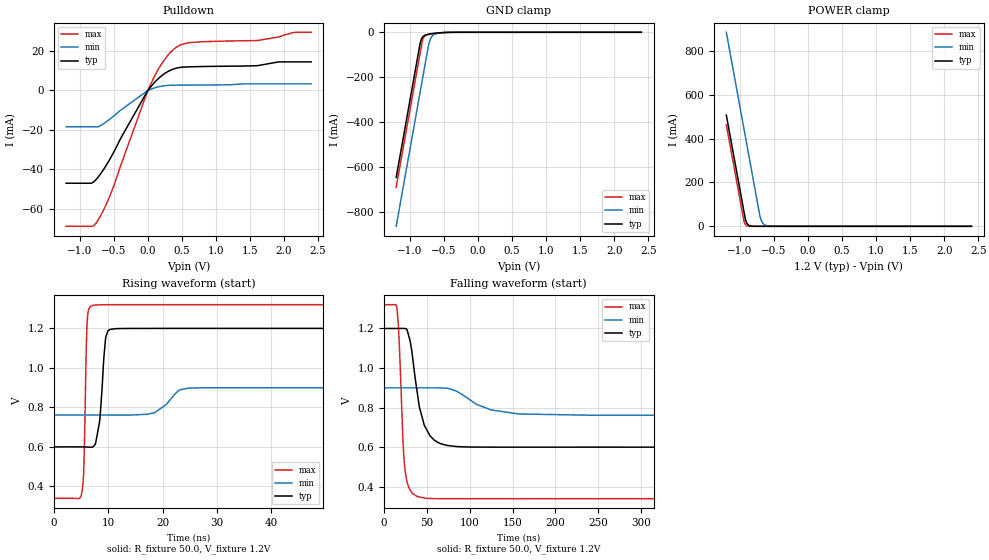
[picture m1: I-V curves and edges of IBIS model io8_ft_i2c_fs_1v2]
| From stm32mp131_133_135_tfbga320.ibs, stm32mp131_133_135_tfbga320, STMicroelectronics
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|   io8_ft_i2c_fs_1v2
[Model]   io8_ft_i2c_fs_1v2
Model_type I/O_open_drain
Polarity   Non-Inverting
Enable   Active-Low
| CAP_THRESHOLD on pad IOFT is "UDTCAPC" :
| Rising=20.0% of vddiom   Falling=80.0% of vddiom
| C_comp min and max val. don't necessarily correlate with the min and max pvt
| but are the smallest and greatest pad capacitance found.
| var   typ   min   max
C_comp   1.36950pF  1.28335pF  1.45130pF
Vinl = 360.0mV
Vinh = 840.0mV
Vmeas = 600.0mV   | Reference voltage for timing measurements
Cref  = 100.0nF   | Timing specification test load capacitance value
Rref  = 1.0kOhm   | Timing specification test load resistance value
Vref  = 600.1mV   | Timing specification test load voltage
[Model Spec]
| TIME_THRESHOLD on pin ZIV11 is "CMOS" :
| Rising=40.0% of vdd   Falling=60.0% of vdd
Vinl 465.80000mV 358.80000mV 518.80000mV
Vinh 741.20000mV 543.20000mV 820.20000mV
| variable   typ   min   max
[Temperature Range] 25.0 140.0 -40.0
| variable   typ   min   max
[Voltage Range] 1.2V 900.0mV 1.32V
| variable   typ   min   max
[POWER Clamp Reference] 1.2V 900.0mV 1.32V
| variable   typ   min   max
[GND Clamp Reference] 0V 0V 0V
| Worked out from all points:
|   slope of the pulldown table from 0 to 0.18 V, typ, clamps not added: 26.5 ohm
|   GND clamp passes 1 mA (typ) near -0.49 V on its own axis
|   POWER clamp passes 1 mA (typ) near -0.83 V on its own axis
|   rising waveform, R_fixture 50.0, V_fixture 1.2V: 20-80 % time 927ps typ, 3.09ns min, 434ps max; typ from 0.6 V to 1.2 V
|   falling waveform, R_fixture 50.0, V_fixture 1.2V: 20-80 % time 13.8ns typ, 35.7ns min, 5.62ns max; typ from 1.2 V to 0.6 V
[POWER Clamp]
-1.2V     507mA      884.8mA    462.5mA
-950mV    82mA       459.8mA    37.51mA
-930mV    48mA       425.8mA    13.86mA
-910mV    22.04mA    391.8mA    5.123mA
-890mV    10.12mA    357.8mA    1.893mA
-870mV    4.646mA    323.8mA    699.7uA
-710mV    9.171uA    51.95mA    243.5nA
-680mV    2.852uA    22.37mA    54.74nA
-650mV    886.6nA    9.63mA     12.33nA
-600mV    125.8nA    2.365mA    1.054nA
-490mV    1.049nA    108uA      41.48pA
2.4V      0A         0A         0A
[GND Clamp]
-1.2V     -646.3mA   -864.2mA   -690.1mA
-850mV    -51.35mA   -269.2mA   -95.05mA
-840mV    -39.26mA   -252.2mA   -78.05mA
-820mV    -24.85mA   -218.2mA   -44.05mA
-800mV    -17.5mA    -184.2mA   -25.22mA
-770mV    -12.13mA   -133.2mA   -15.02mA
-720mV    -8.143mA   -50.86mA   -9.665mA
-690mV    -6.656mA   -25.2mA    -7.855mA
-660mV    -5.424mA   -13.63mA   -6.324mA
-570mV    -2.602mA   -3.787mA   -2.765mA
-350mV    -41.28uA   -263.5uA   -8.566uA
2.4V      4.788nA    1.261uA    272.6pA
| variable   typ   min   max
[Pullup Reference] 1.2V 900.0mV 1.32V
| variable   typ   min   max
[Pulldown Reference] 0V 0V 0V
[Pulldown]
-1.2V     -47.11mA   -18.46mA   -68.98mA
-810mV    -46.78mA   -18.46mA   -68.93mA
-730mV    -44.02mA   -18.46mA   -65.79mA
-630mV    -39.07mA   -16.4mA    -59.3mA
-530mV    -33.22mA   -13.8mA    -51.19mA
0V        0A         0A         1fA
200mV     7.375mA    2.155mA    13.36mA
390mV     11.04mA    2.691mA    21.16mA
600mV     11.99mA    2.746mA    24.23mA
1.61V     12.59mA    3.342mA    25.35mA
2.15V     14.51mA    3.342mA    29.49mA
2.4V      14.51mA    3.342mA    29.54mA
[Ramp]
dV/dt_r 359.77616mV/926.94531ps 83.02607mV/3.08575ns 587.93904mV/432.99808ps
dV/dt_f 359.70168mV/13.79478ns 83.0117mV/35.69932ns 587.93923mV/5.62319ns
R_load = 50.0
| Removed startup time: 0s 0s 0s  .
| Removed end time: 2.1994us.
[Rising Waveform]
R_fixture   = 50.0
V_fixture   = 1.2V
V_fixture_min = 900.0mV
V_fixture_max = 1.32V
0s        600.4mV    761.6mV    340.1mV
5.1ns     600.3mV    761.6mV    362.6mV
5.5ns     600.2mV    761.6mV    474.1mV
6.2ns     599.2mV    761.6mV    1.261V
7.7ns     620.6mV    761.6mV    1.318V
8.8ns     866.8mV    761.6mV    1.319V
9.9ns     1.184V     761.5mV    1.32V
14.2ns    1.2V       761.5mV    1.32V
28.6ns    1.2V       899.6mV    1.32V
2.199us   1.2V       900mV      1.32V
| Removed startup time: 0s 0s 0s  .
| Removed end time: 2.1994us.
[Falling Waveform]
R_fixture   = 50.0
V_fixture   = 1.2V
V_fixture_min = 900.0mV
V_fixture_max = 1.32V
0s        1.2V       900mV      1.32V
14.8ns    1.2V       900mV      1.313V
17ns      1.2V       900mV      1.202V
23ns      1.2V       900mV      565.9mV
26.7ns    1.196V     900mV      430.2mV
48.6ns    698.3mV    900mV      341.9mV
85.2ns    603.3mV    882.3mV    340.1mV
125.3ns   600.5mV    788.3mV    340.1mV
244.4ns   600.5mV    761.6mV    340.1mV
2.199us   600.5mV    761.6mV    340.1mV
